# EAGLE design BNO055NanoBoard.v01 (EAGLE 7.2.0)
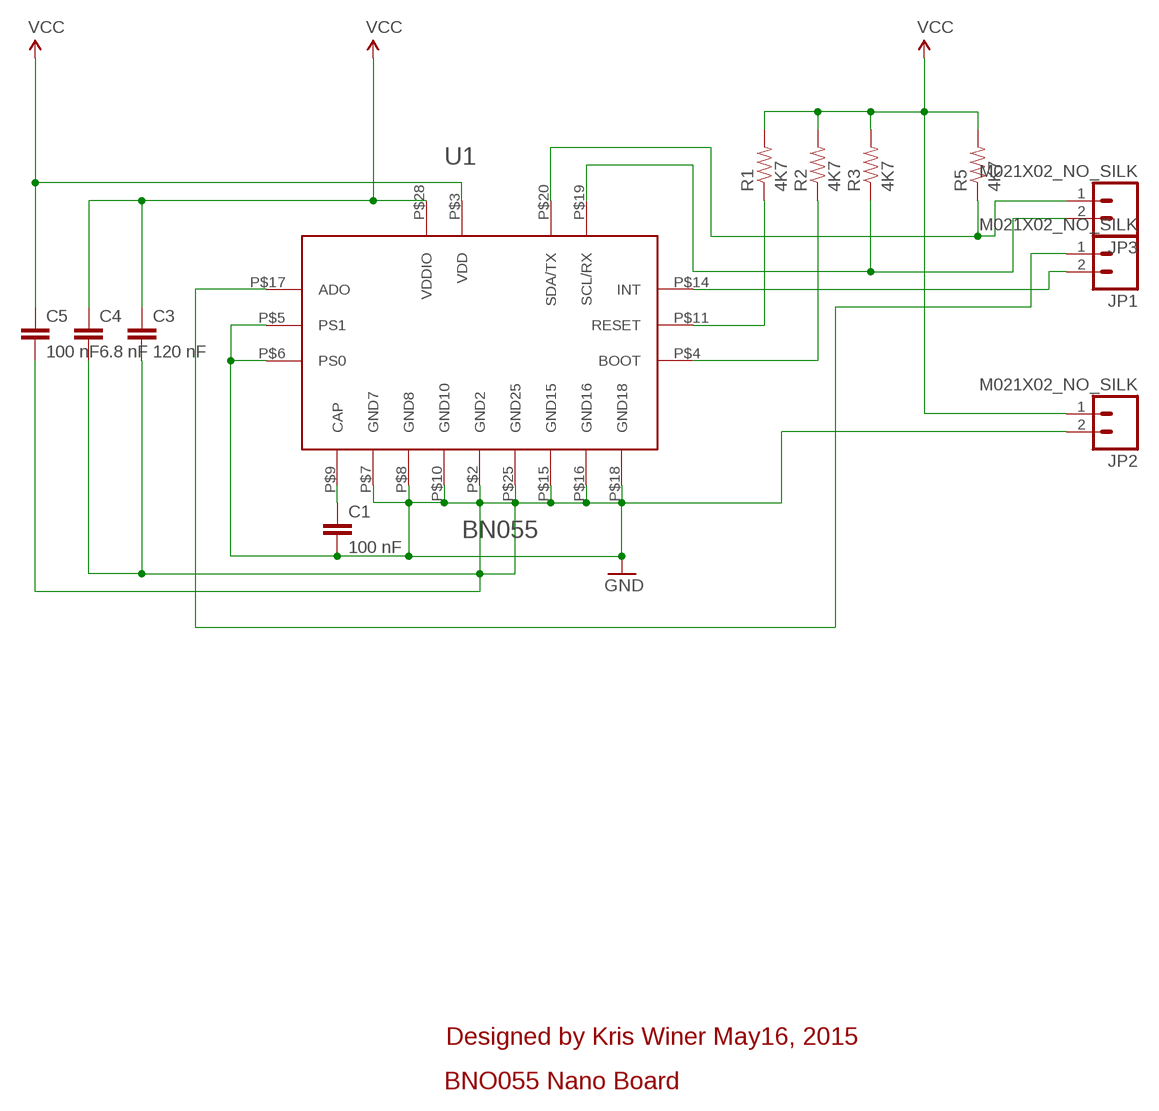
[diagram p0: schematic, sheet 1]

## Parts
C1  100 nF  CAP0402-CAP  [0402-CAP]
C3  120 nF  CAP0402-CAP  [0402-CAP]
C4  6.8 nF  CAP0402-CAP  [0402-CAP]
C5  100 nF  CAP0402-CAP  [0402-CAP]
JP1  M021X02_NO_SILK  [1X02_NO_SILK]
JP2  M021X02_NO_SILK  [1X02_NO_SILK]
JP3  M021X02_NO_SILK  [1X02_NO_SILK]
R1  4K7  RESISTOR0402-RES  [0402-RES]
R2  4K7  RESISTOR0402-RES  [0402-RES]
R3  4K7  RESISTOR0402-RES  [0402-RES]
R5  4K7  RESISTOR0402-RES  [0402-RES]
U1  BN055  [LGA28]

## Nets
GND: C1.2 C3.2 C4.2 C5.2 JP2.2 U1.P$2(GND2) U1.P$5(PS1) U1.P$6(PS0) U1.P$7(GND7) U1.P$8(GND8) U1.P$10(GND10) U1.P$15(GND15) U1.P$16(GND16) U1.P$18(GND18) U1.P$25(GND25)
N$1: JP1.2 U1.P$14(INT)
N$2: R1.1 U1.P$11(RESET)
N$3: C1.1 U1.P$9(CAP)
N$4: JP1.1 U1.P$17(ADO)
N$6: R2.1 U1.P$4(BOOT)
SCL: JP3.2 R3.1 U1.P$19(SCL/RX)
SDA: JP3.1 R5.1 U1.P$20(SDA/TX)
VCC: C3.1 C4.1 C5.1 JP2.1 R1.2 R2.2 R3.2 R5.2 U1.P$3(VDD) U1.P$28(VDDIO)

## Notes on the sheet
- Designed by Kris Winer May16, 2015
- BNO055 Nano Board

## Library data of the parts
C1 C3-C5 = SparkFun-Capacitors:CAP: Capacitor
JP1-JP3 = SparkFun-Connectors:M02: Standard 2-pin 0.1" header. Use with
R1-R3 R5 = SparkFun-Passives:RESISTOR: Resistor
U1 = SparkFun-DigitalIC:BN055

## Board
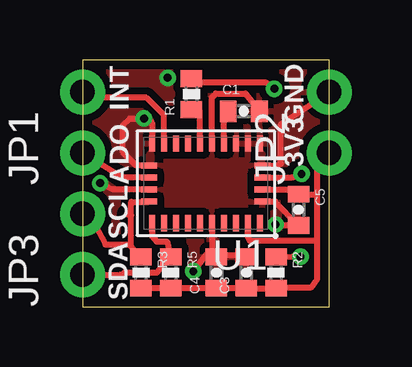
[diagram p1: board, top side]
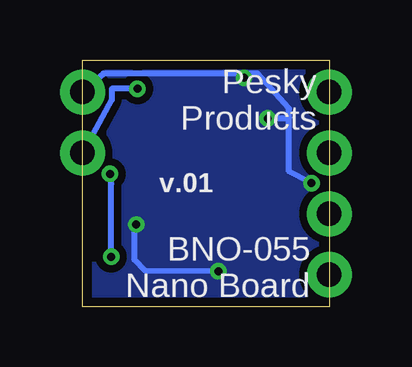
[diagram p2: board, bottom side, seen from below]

Size 10.29 x 10.29 mm. Coordinates in mm from the lower left corner, seen from the top.
Outline: 0,0 10.29,0 10.29,10.29 0,10.29 0,0
Copper layers (1*16): Top 0.0356mm / dielectric 1.5011mm / Bottom 0.0356mm
Design rules "OSHPark *": minimum track width 6mil, minimum drill 13mil, track to track 6mil, track to pad 6mil, pad to pad 6mil, via to via 6mil, smd to smd 6mil, copper to edge 15mil, drill to drill 6mil, minimum pad ring 7mil, minimum via ring 7mil, stop-mask expansion 3mil, vias tented up to drill 20mil, thermal gap 10mil

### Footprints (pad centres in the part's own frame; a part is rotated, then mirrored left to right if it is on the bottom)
0402-CAP = smd 0.7 x 0.9: 1 -0.65,0; 2 0.65,0
1X02_NO_SILK = drill 1.016 pad 1.88: 1 0,0; 2 2.54,0
0402-RES = smd 0.7 x 0.9: 1 -0.65,0; 2 0.65,0
LGA28 = smd 0.25 x 0.675: P$1 -2.25,1.663; P$6 -2.25,-1.663; P$7 -1.75,-1.663; P$8 -1.25,-1.663; P$9 -0.75,-1.663; P$10 -0.25,-1.663; P$11 0.25,-1.663; P$12 0.75,-1.663; P$13 1.25,-1.663; P$14 1.75,-1.663; P$15 2.25,-1.663; P$20 2.25,1.663; P$21 1.75,1.663; P$22 1.25,1.663; P$23 0.75,1.663; P$24 0.25,1.663; P$25 -0.25,1.663; P$26 -0.75,1.663; P$27 -1.25,1.663; P$28 -1.75,1.663 | smd 0.675 x 0.25: P$2 -2.362,0.75; P$3 -2.362,0.25; P$4 -2.362,-0.25; P$5 -2.362,-0.75; P$16 2.362,-0.75; P$17 2.362,-0.25; P$18 2.362,0.25; P$19 2.362,0.75

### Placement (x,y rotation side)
C1  6.73,8.15 0 top
C3  6.83,1.42 90 top
C4  5.59,1.42 90 top
C5  9.02,4.04 270 top
JP1  0,6.41 90 top
JP2  10.29,6.41 90 top
JP3  0,1.33 90 top
R1  4.55,8.86 90 top
R2  8.08,1.42 270 top
R3  2.44,1.42 270 top
R5  3.68,1.42 270 top
U1  5.15,5.15 180 top

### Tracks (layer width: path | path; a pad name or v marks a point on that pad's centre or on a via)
GND  (via drill 0.33)
  Top 0.254: U1.P$2 8.03,4.4 C5.2 7.96,3.39 v8.05,3.43 | U1.P$5 8.11,5.9 8.28,5.97 8.28,7.63 JP2.2 | U1.P$18 1.24,4.9 v0.74,5.16 | U1.P$15 2.9,7.67 2.72,7.85 v2.56,7.85 1.98,7.85 1.68,7.54 1.68,6.45 2.23,5.9 U1.P$16 | C1.2 6.8,8.89 5.56,8.89 5.4,8.72 U1.P$10 | v4.62,1.47 5.16,2.16 5.4,2.16 | U1.P$25 5.4,2.16 | 5.4,2.16 C4.2 | 5.4,2.16 6.75,2.16 C3.2
  Bottom 0.254: v0.74,5.16 1.68,5.64 1.68,7.87 | 1.68,7.87 1.68,8.26 3,9.73 9.42,9.73 JP2.2 | v2.56,7.85 1.7,7.85 1.68,7.87 | v4.62,1.47 7.67,1.5 8.13,1.96 8.13,3.35 v8.05,3.43 8.03,3.45
  other vias: 3.56,9.55
  pour Top (isolate 0.305): 0,10.29 10.29,10.29 10.29,0 0,0
  pour Bottom (isolate 0.305): 0,10.29 10.29,10.29 10.29,0 0,0
N$1
  Top 0.254: U1.P$14 3.4,7.98 2.67,8.71 0.24,8.71 JP1.2
N$2
  Top 0.254: U1.P$11 4.9,8.17 R1.1
N$3
  Top 0.254: U1.P$9 5.9,8.22 C1.1
N$4
  Top 0.254: U1.P$17 1.65,5.4 JP1.1
N$6  (via drill 0.33)
  Top 0.254: R2.1 8.8,2.1 v9.09,2.08 | U1.P$4 8.72,5.4 v9.14,5.54
  Bottom 0.254: v9.09,2.08 9.09,5.13 v9.14,5.54
SCL
  Top 0.254: R3.1 2.37,2.07 2.03,2.52 | 2.03,2.52 2.03,3.81 | 2.03,3.81 2.03,4.37 2.76,4.37 U1.P$19 | 1.87,3.87 2.03,3.81 | JP3.2 0.28,3.86 0.96,2.59 1.85,2.59 2.03,2.52
SDA
  Top 0.254: U1.P$20 2.9,2.94 3.1,2.72 3.52,2.72 R5.1 3.11,1.42 1.75,1.42 1.59,1.33 JP3.1
VCC  (via drill 0.33)
  Top 0.254: U1.P$3 8.99,4.9 C5.1 9.76,4.69 9.78,4.78 | 6.9,3.04 U1.P$28 6.91,2.9 6.99,2.74 9.78,2.74 | R3.2 R5.2 C4.1 C3.1 6.64,0.74 7.9,0.74 7.95,0.79 R2.2 7.96,0.79 9.53,0.79 9.78,1.14 9.78,2.74 | 9.78,4.78 9.78,2.74 | JP2.1 10.04,6.43 9.78,5.79 9.78,4.78 | v8,9.09 7.68,9.34 4.72,9.34 R1.2
  Bottom 0.254: v8,9.09 9.07,9.09 9.07,8.63 JP2.1

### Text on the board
tPlace: INT | GND | ADO | 3V3 | SCL | SDA
bPlace: Pesky / Products | v.01 | BNO-055 / Nano Board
